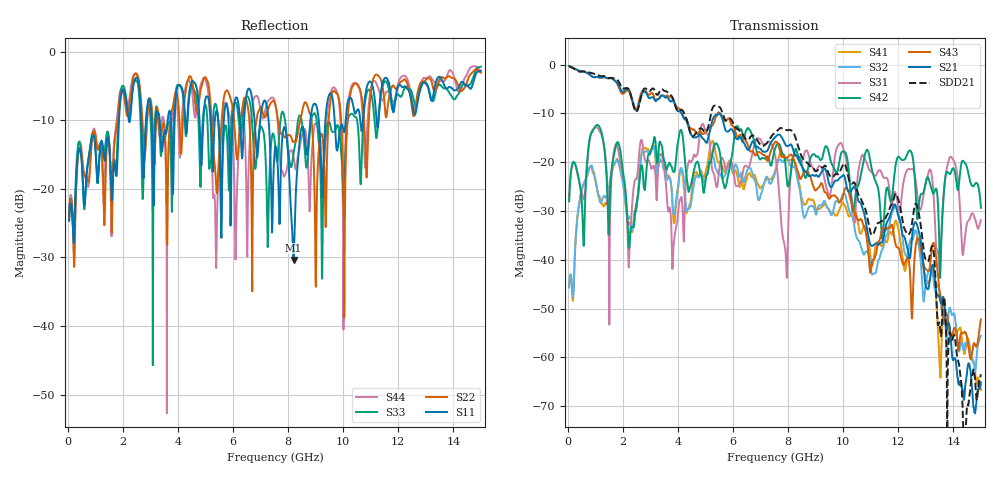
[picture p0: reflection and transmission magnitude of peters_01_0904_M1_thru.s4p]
# MHZ S RI R 50.00
! FREQ  S11  S12  S13  S14
!  S21  S22  S23  S24
!  S31  S32  S33  S34
!  S41  S42  S43  S44
!  REAL  IMAG  REAL  IMAG  REAL  IMAG  REAL  IMAG
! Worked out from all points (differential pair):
!   1496 points, 50 MHz to 15 GHz, reference 50 ohm
!   strongest paths, dB at 50 MHz, 3.79 GHz, 7.53 GHz, 11.27 GHz, 15 GHz:
!     S21: -0.3, -7.4, -14.9, -36.9, -65.1
!     S43: -0.3, -6.9, -15.9, -36.5, -52.2
!     S42: -28.0, -21.2, -17.2, -25.5, -29.3
!     S31: -28.0, -40.0, -18.7, -21.8, -31.9
!     S32: -45.7, -27.3, -22.1, -40.2, -55.6
!     S41: -45.6, -27.1, -21.8, -36.4, -66.4
!   taken as a pair (ports 1,3 in; 2,4 out), SDD21 dB: -0.3, -6.6, -14.0, -32.4, -63.5
!   lowest |S11| = -30.4 dB at 8.2 GHz (marker M1), VSWR 1.06, Z = 47.4 + j1.43 ohm
!   |S11| at or under -10 dB: start of sweep to 1.861 GHz; 7.292 GHz to 8.811 GHz (1.519 GHz wide, 18.9 % of centre); 9.69 GHz to 10.09 GHz (401.9 MHz wide, 4.06 % of centre)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
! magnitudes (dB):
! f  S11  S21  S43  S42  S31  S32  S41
! 50 MHz  -24.7  -0.3  -0.3  -28.0  -28.0  -45.7  -45.6
! 820 MHz  -13.9  -2.1  -2.2  -14.6  -14.7  -20.8  -21.1
! 3.84 GHz  -17.2  -7.5  -7.3  -22.0  -37.3  -30.4  -32.1
! 4.89 GHz  -13.2  -15.0  -14.2  -24.2  -12.2  -23.2  -22.6
! 7.92 GHz  -11.7  -16.5  -19.1  -21.4  -39.4  -19.3  -19.3
! 8.2 GHz  -30.4  -17.7  -19.5  -18.7  -18.7  -20.9  -19.3
! 15 GHz  -2.8  -65.1  -52.2  -29.3  -31.9  -55.6  -66.4
